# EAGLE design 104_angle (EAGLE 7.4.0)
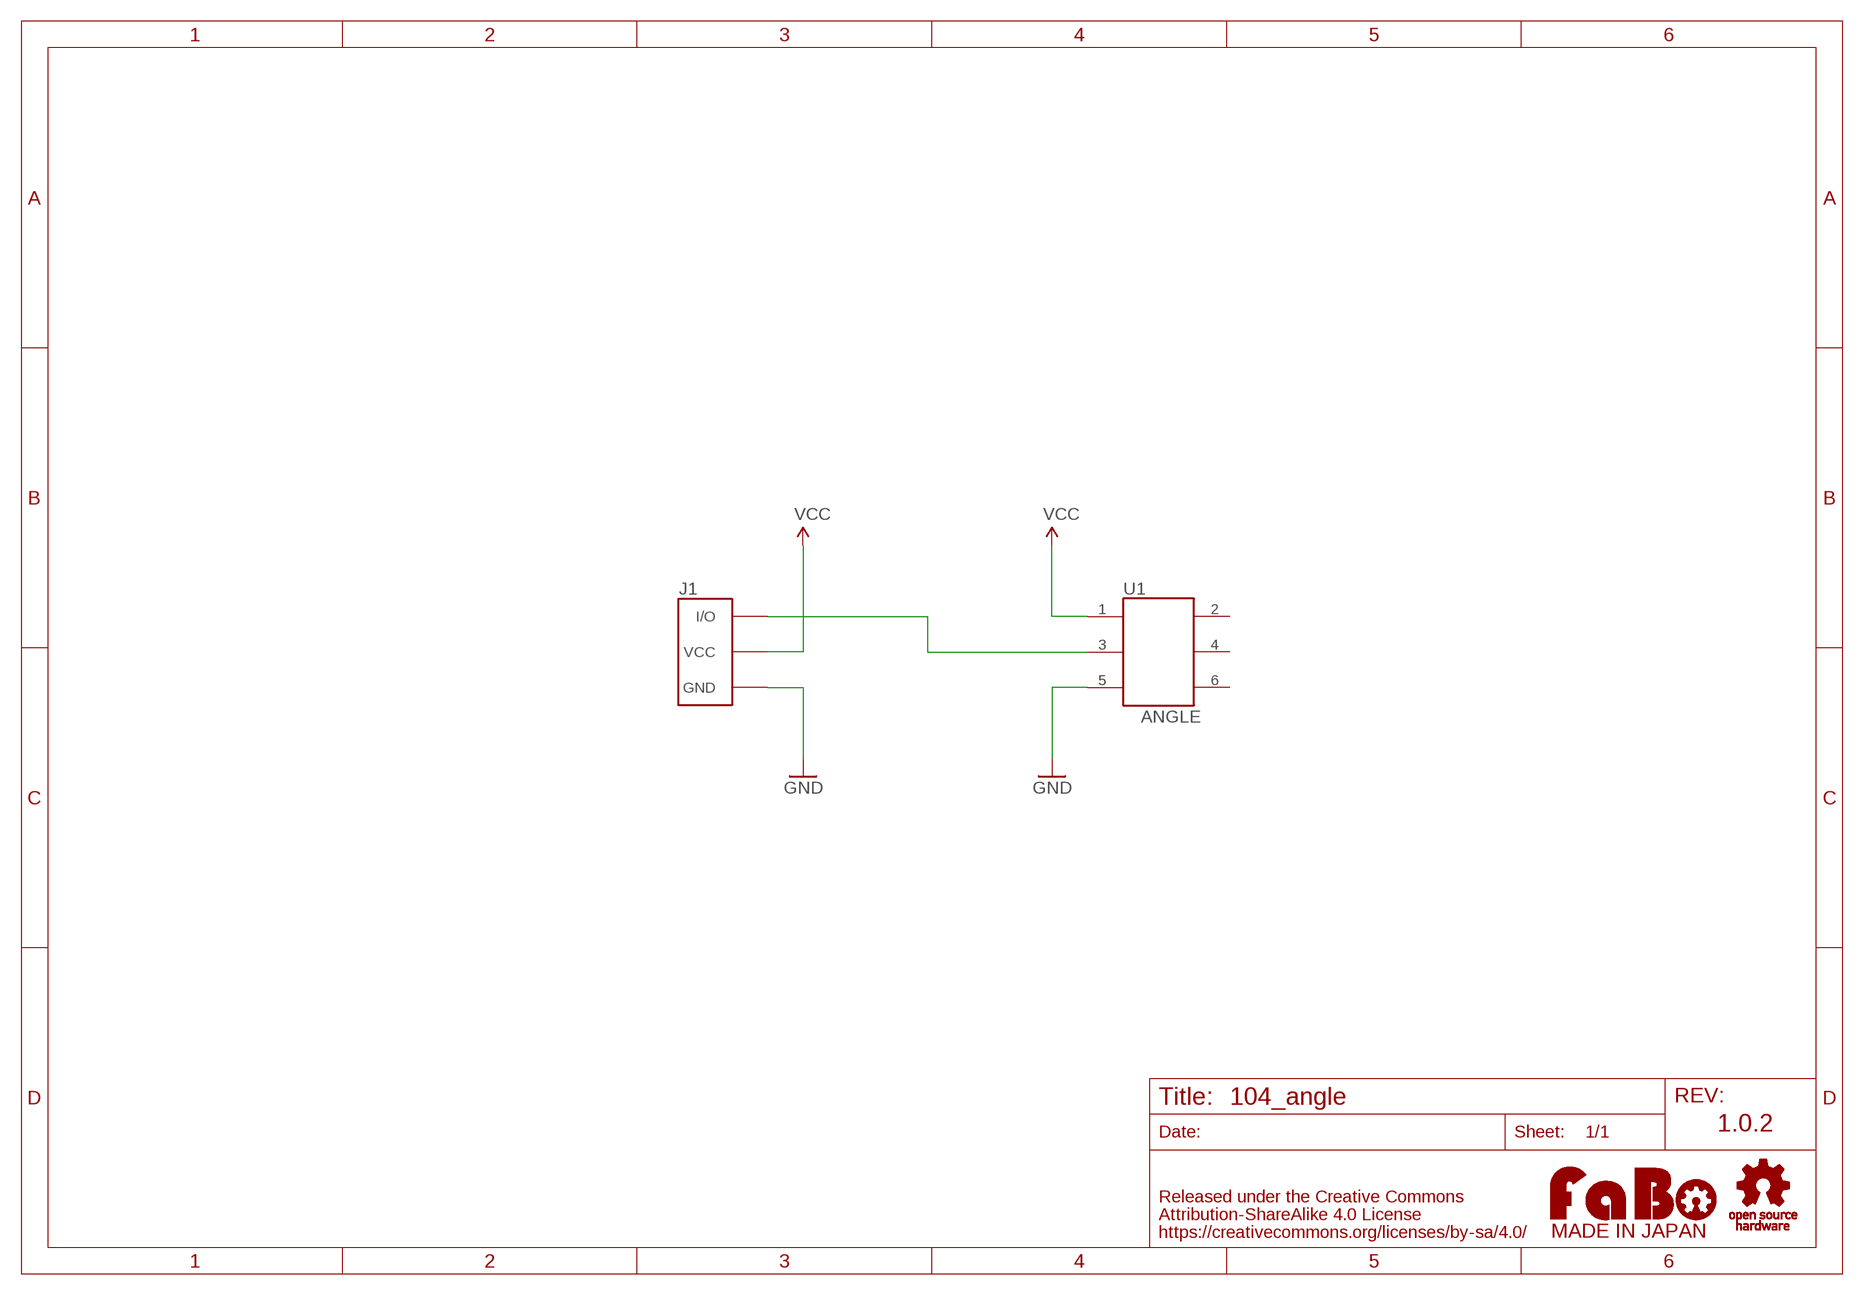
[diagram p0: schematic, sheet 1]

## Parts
J1  FABO_BRICK_3PIN  [FABO_BRICK_3PIN]
U1  ANGLE  ROTARYENCORDER_BRICK  [ROTARYENCORDER_BRICK]
U$2  LOGO_FABO-M  [LOGO_FABO_MS]
U$3  LOGO_OSHW-T_M_BOTTOM  [LOGO_OSHW_T_MS_BOTTOM]

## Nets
GND: J1.GND U1.5
N$1: J1.IN/OUT(I/O) U1.3
VCC: J1.VCC U1.1
Unconnected: U1.2 U1.4 U1.6

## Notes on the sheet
- 1.0.2

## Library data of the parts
J1 = FaBo-Template:FABO_BRICK_3PIN: FaBo Brick 3pin
U1 = FaBo-etc:ROTARYENCORDER_BRICK: Rotary Encorder for Brick
U$2 = FaBo-etc:LOGO_FABO
U$3 = FaBo-etc:LOGO_OSHW

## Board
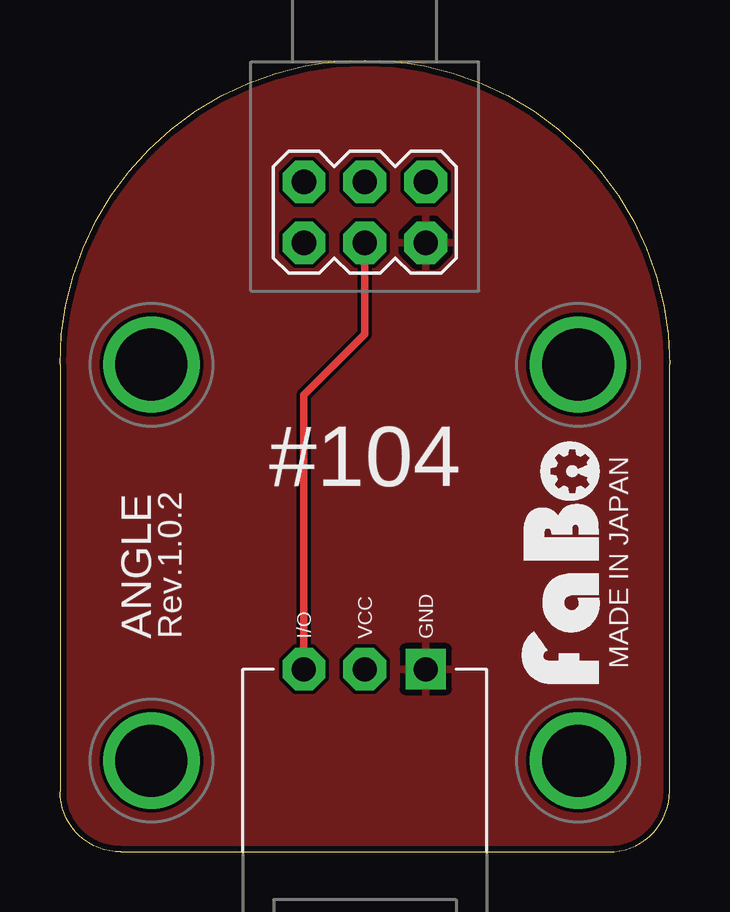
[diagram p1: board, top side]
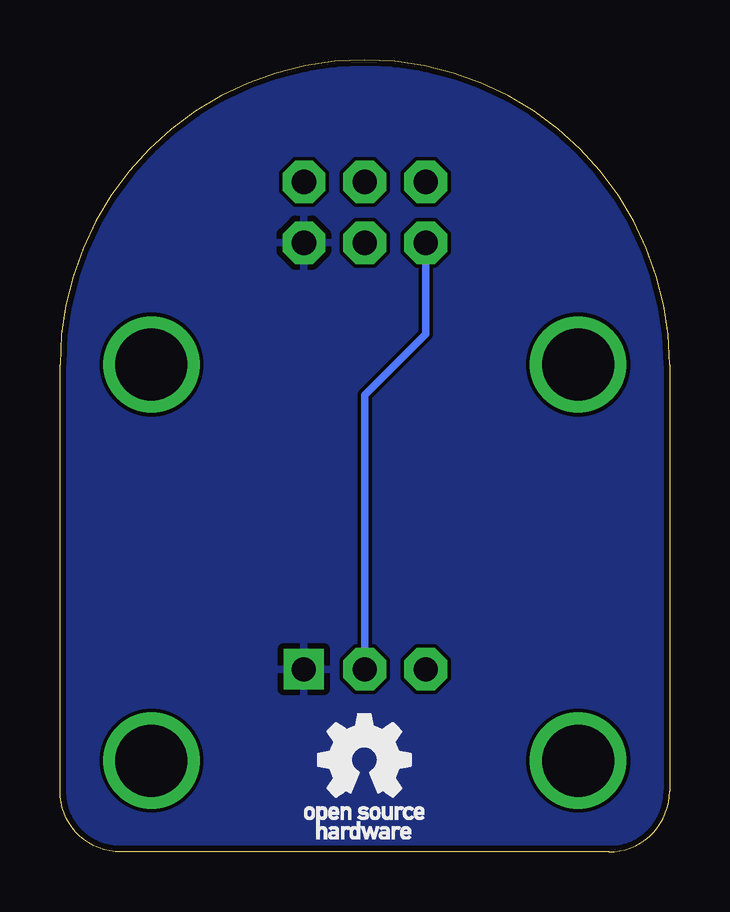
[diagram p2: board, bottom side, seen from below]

Size 25.4 x 33.02 mm. Coordinates in mm from the lower left corner, seen from the top.
Copper layers (1*16): Top 0.035mm / dielectric 1.5mm / Bottom 0.035mm
Design rules "Elecrow_2-layer_eagle_rule": minimum track width 6mil, minimum drill 12mil, track to track 6mil, track to pad 6mil, pad to pad 6mil, via to via 6mil, smd to smd 0mil, copper to edge 10mil, drill to drill 10mil, minimum pad ring 10mil, minimum via ring 6mil, stop-mask expansion 2mil, vias tented up to drill 100mil, thermal gap 10mil

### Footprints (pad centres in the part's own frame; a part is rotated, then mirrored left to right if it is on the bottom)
FABO_BRICK_3PIN = drill 1 pad 1.676 square: GND 2.54,-8.89 | drill 1 pad 1.778 octagon: IN/OUT -2.54,-8.89; VCC 0,-8.89 | drill 3 pad 3.81: P$5 -8.89,3.81; P$6 8.89,3.81; P$7 -8.89,-12.7; P$8 8.89,-12.7
ROTARYENCORDER_BRICK = drill 1.016 pad 1.778 octagon: 1 -2.54,-1.27; 2 -2.54,1.27; 3 0,-1.27; 4 0,1.27; 5 2.54,-1.27; 6 2.54,1.27

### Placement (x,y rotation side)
J1  12.7,16.51 0 top
U1  12.7,26.67 0 top
U$2  22.86,12.06 90 top
U$3  12.7,3.81 0 top

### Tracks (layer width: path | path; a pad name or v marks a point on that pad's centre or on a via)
GND
  pour Bottom: -1.27,-1.27 26.67,-1.27 26.67,34.29 -1.27,34.29
  pour Top: -1.27,-1.27 26.67,-1.27 26.67,34.29 -1.27,34.29
N$1
  Top 0.305: U1.3 12.7,21.59 10.16,19.05 J1.IN/OUT
VCC
  Bottom 0.305: U1.1 10.16,21.59 12.7,19.05 J1.VCC

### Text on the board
tPlace: #104 | MADE IN JAPAN | ANGLE | Rev.1.0.2

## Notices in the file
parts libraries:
FaBo-etc: Released under the Creative Commons Attribution-ShareAlike 4.0 License
https://creativecommons.org/licenses/by-sa/4.0
FaBo-etc: Released under the Creative Commons
